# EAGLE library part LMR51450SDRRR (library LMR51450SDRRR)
Switching Voltage Regulators 36-V, 5-A synchronous buck converter Source: Datasheet
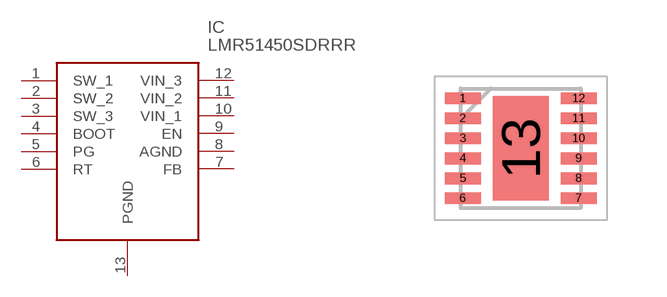
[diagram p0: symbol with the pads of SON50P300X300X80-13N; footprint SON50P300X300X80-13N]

Designator prefix IC

## LMR51450SDRRR (Description: Switching Voltage Regulators 36-V, 5-A synchronous buck converter; Height: 0.8mm; Manufacturer_Name: Texas Instruments; Manufacturer_Part_Number: LMR51450SDRRR; Mouser_Part_Number: 595-LMR51450SDRRR; Mouser_Price-Stock: https://www.mouser.co.uk/ProductDetail/Texas-Instruments/LMR51450SDRRR?qs=rQFj71Wb1eUvKinsjoLiUA%3D%3D)  [SON50P300X300X80-13N]
1  SW_1
2  SW_2
3  SW_3
4  BOOT
5  PG
6  RT
7  FB
8  AGND
9  EN
10  VIN_1
11  VIN_2
12  VIN_3
13  PGND

## Footprint SON50P300X300X80-13N (pad centres in mm)
DRR0012G
smd 0.9 x 0.3: 1 -1.45,1.25; 2 -1.45,0.75; 3 -1.45,0.25; 4 -1.45,-0.25; 5 -1.45,-0.75; 6 -1.45,-1.25; 7 1.45,-1.25; 8 1.45,-0.75; 9 1.45,-0.25; 10 1.45,0.25; 11 1.45,0.75; 12 1.45,1.25
smd 1.4 x 2.6: 13 0,0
